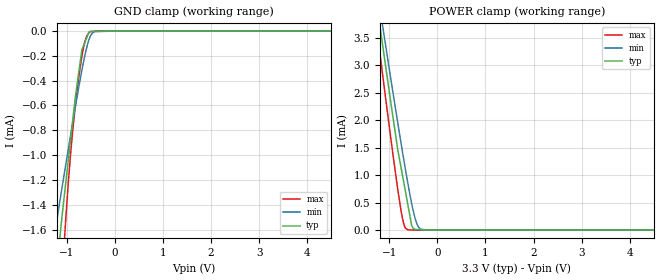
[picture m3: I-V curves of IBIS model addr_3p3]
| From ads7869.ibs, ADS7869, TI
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|   addr_3p3 Model
[Model]   addr_3p3
Model_type   Input
Vinl = 0.8
Vinh = 2.0
|   typ   min   max
|   (nom PVT)   (fast PVT)   (slow PVT)
|C_comp from frequency sweep method (F=8MHz)
|Average
|C_comp   2.334e-12   2.248e-12   2.420e-12
|C_comp from LC tank measurement(L=1nH)
|Average
|Resonant Frequency(Hz)   3.590e+09   3.640e+09   3.530e+09
C_comp   1.967e-12   1.914e-12   2.035e-12
| Where nom  PVT is Nominal Process, 3.3V, 36C
|   Fast PVT is Strong Process,  3.6V, -40C
|   Slow PVT is Weak Process,   3V, 96C
[Voltage Range]   3.3   3   3.6
|Ambient Temperature   25   85   -40
|Junction Temperature
[Temperature Range]   36   96   -40
[Power Clamp Reference]   3.3   3   3.6
[GND Clamp Reference]   0   0   0
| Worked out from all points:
|   GND clamp passes 1 mA (typ) near -0.96 V on its own axis
|   POWER clamp passes 1 mA (typ) near -0.73 V on its own axis
[GND Clamp]
|   Voltage   I(typ)   I(min)   I(max)
-3.3V     -9.858mA   -6.77mA    -17.28mA
-1.374V   -2.514mA   -1.934mA   -3.774mA
-1.14V    -1.645mA   -1.359mA   -2.241mA
-1.096V   -1.48mA    -1.253mA   -1.968mA
-1.025V   -1.234mA   -1.084mA   -1.532mA
-877.2mV  -720.8uA   -736.1uA   -803.8uA
-686.4mV  -150uA     -316uA     -203.8uA
-614.4mV  -81.38uA   -179.7uA   -71.1uA
-534.6mV  -5.332uA   -64.01uA   -11.71uA
-414mV    -2.63uA    -3.831uA   -759.4nA
-28.87fV  0A         0A         0A
6.6V      0A         0A         0A
[POWER Clamp]
|   Voltage   I(typ)   I(min)   I(max)
-3.3V     17.16mA    16.43mA    18.25mA
-1.259V   4.122mA    4.413mA    3.661mA
-1.167V   3.545mA    3.881mA    3.025mA
-1.135V   3.346mA    3.7mA      2.805mA
-825mV    1.469mA    1.956mA    743.9uA
-754.8mV  1.133mA    1.577mA    345.2uA
-679.2mV  771.9uA    1.18mA     57.25uA
-610.8mV  444.9uA    835uA      2.249uA
-531.3mV  73.95uA    465.9uA    475.3nA
-426mV    7.712uA    109.1uA    0A
-339mV    5.681uA    11.41uA    0A
6.6V      0A         0A         0A
